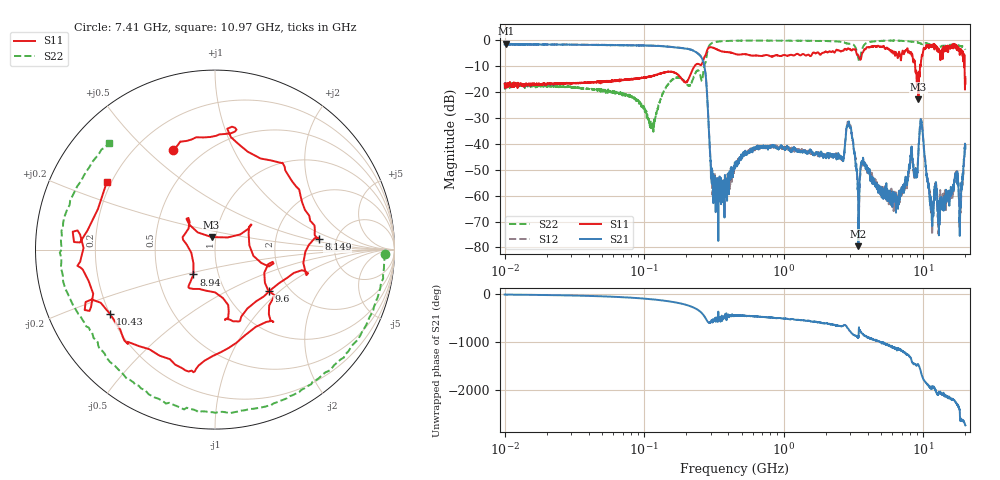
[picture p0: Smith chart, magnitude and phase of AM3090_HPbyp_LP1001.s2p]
# Hz S DB R 50
!freq MagS11 AngS11 MagS21 AngS21 MagS12 AngS12 MagS22 AngS22
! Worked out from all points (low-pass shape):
!   3201 points, 10 MHz to 20 GHz, reference 50 ohm
!   highest |S21| = -1.45 dB at 10.19 MHz (marker M1); lowest = -79.5 dB at 3.424 GHz (marker M2)
!   |S21| within 3 dB of the highest: start of sweep to 230.4 MHz
!   lowest |S11| = -22.8 dB at 9.22 GHz (marker M3), VSWR 1.16, Z = 47.7 + j6.69 ohm
!   |S11| at or under -10 dB: start of sweep to 230.1 MHz; 8.73 GHz to 9.466 GHz (735.5 MHz wide, 8.08 % of centre); 19.73 GHz to end of sweep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
!   |S22| runs from -35.4 to -0.2 dB; largest |S21 - S12| = 0.033
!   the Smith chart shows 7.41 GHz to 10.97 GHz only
!   S11 on the Smith chart (normalised r, x): 7.41 GHz: 0.35, +0.61; 8.149 GHz: 3.64, +0.63; 8.94 GHz: 0.76, -0.22; 9.6 GHz: 1.57, -0.85; 10.43 GHz: 0.20, -0.27; 10.97 GHz: 0.18, +0.28
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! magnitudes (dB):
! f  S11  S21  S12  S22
! 10 MHz  -16.9  -1.8  -1.5  -17.0
! 10.19 MHz  -18.3  -1.5  -1.8  -18.1
! 35.55 MHz  -16.5  -1.9  -1.9  -18.6
! 126.1 MHz  -13.2  -2.3  -2.3  -26.0
! 254.1 MHz  -9.7  -6.3  -6.2  -14.5
! 274.8 MHz  -5.9  -12.9  -12.7  -8.7
! 313.9 MHz  -3.1  -54.3  -55.2  -1.0
! 447.2 MHz  -5.4  -49.6  -47.7  -0.3
! 1.59 GHz  -5.6  -43.5  -43.7  -0.3
! 2.612 GHz  -4.2  -45.5  -45.8  -0.8
! 2.914 GHz  -3.3  -31.5  -32.2  -1.5
! 3.424 GHz  -6.1  -79.5  -63.8  -7.3
! 5.639 GHz  -3.7  -61.8  -60.0  -0.3
! 7.41 GHz  -4.4  -54.2  -55.6  -0.5
! 8.149 GHz  -4.7  -42.7  -44.9  -0.7
! 8.94 GHz  -14.7  -51.3  -51.7  -0.8
! 9.22 GHz  -22.8  -42.5  -42.9  -1.0
! 9.6 GHz  -8.5  -30.8  -31.3  -1.5
! 10.43 GHz  -3.3  -49.1  -48.8  -1.3
! 10.97 GHz  -3.0  -55.7  -57.3  -1.6
! 18.4 GHz  -3.5  -62.3  -62.5  -2.4
! 20 GHz  -14.4  -41.9  -40.1  -3.8
